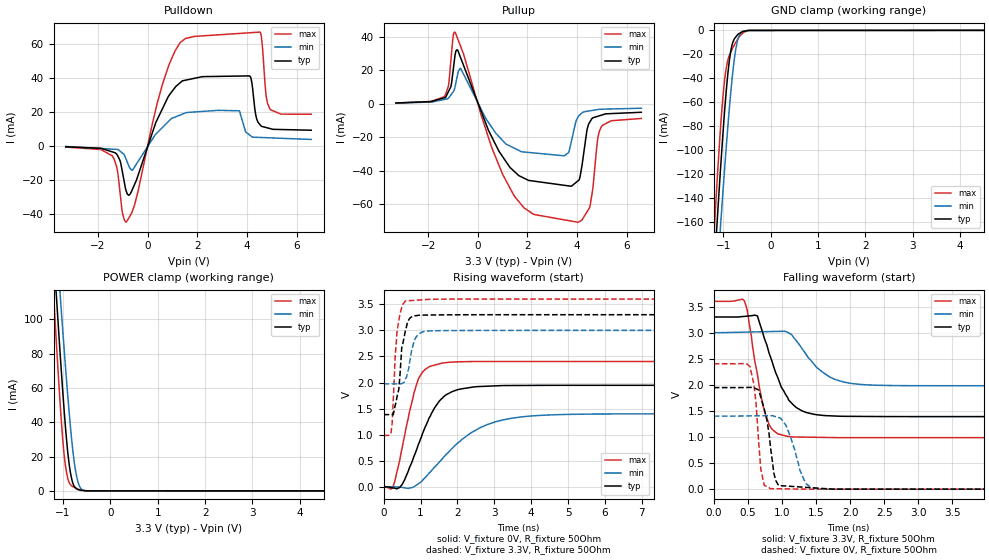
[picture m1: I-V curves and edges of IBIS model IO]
| Texas Instruments Incorporated
| 10-Channel Sequencer and System Health Monitor
| Marketing part#   Voltage Range   Package-type   #pins/pkg drawing
| UCD9090RGZR   3.0V - 3.6V   VQFN   48-pin  RGC
| UCD9090RGZT   3.0V - 3.6V   VQFN   48-pin  RGC
[IBIS ver]   4.0
[File name]   ucd9090.ibs
[File Rev]   1.0
[Date]   10/04/2016
[Source]   Simulations in SPECTRE
   Texas Instruments Incorporated.
   Analog-eLab, HPA
   12500 TI Blvd
   Dallas, TX -75243
   For Support e-mail: elab_ibis@list.ti.com
[Notes]   Revision History
   Rev 1.0: 10/04/2016
   - Initial version of the model
   - Model based on simulations from Spectre
   - Model not matched to measurements
   - Non-monotonic behavior is as per buffer simulations
   - Buffer [Model]s based on ucd9240.ibs Rev 1.1: 09/29/2010
[Disclaimer] This model is designed as an aid for customers of Texas Instruments.
 TI and its licensors and suppliers make no warranties, either expressed
 or implied, with respect to this  model, including the warranties of
 merchantability or fitness for a particular purpose.
 The model is provided solely on an "as is" basis. The entire risk as to
 its quality and performance is with the customer.
[Copyright] (C)Copyright 2016 Texas Instruments Incorporated.
   All rights reserved.
|   Component UCD9090RGZ
[Component]   UCD9090RGZ
[Manufacturer]  Texas Instruments Incorporated
[Package]   |48-pin VQFN package
|   typ   min   max
R_pkg   0.1229   0.0608   0.1600
L_pkg   1.8455n   1.2923n   2.3934n
C_pkg   0.1920p   0.1668p   0.2592p
[Pin] signal_name   model_name   R_pin   L_pin   C_pin
1   MON1   TERM   0.15085   2.25498n   0.20057p
2   MON2   TERM   0.13802   2.04542n   0.20645p
3   RESETN   TERM   0.12831   1.88923n   0.19375p
4   GPIO1   TERM   0.12256   1.79720n   0.17958p
5   GPIO2   TERM   0.13456   1.98873n   0.18502p
6   GPIO3   TERM   0.13010   1.91761n   0.19072p
7   GPIO4   TERM   0.12331   1.80911n   0.18509p
8   PMBUS_CLK   IO   0.12134   1.77773n   0.18285p
9   PMBUS_DATA   IO   0.12282   1.80149n   0.18453p
10   FPWM1_GPIO5  TERM   0.12680   1.86522n   0.18720p
11   FPWM2_GPIO6  TERM   0.13446   1.98842n   0.19728p
12   FPWM3_GPIO7  TERM   0.14463   2.15518n   0.18661p
13   FPWM4_GPIO8  TERM   0.14322   2.13188n   0.18595p
14   FPWM5_GPIO9  TERM   0.13149   1.93932n   0.19489p
15   FPWM6_GPIO10 TERM   0.12192   1.78462n   0.17983p
16   FPWM7_GPIO11 TERM   0.12141   1.77609n   0.17874p
17   FPWM8_GPIO12 TERM   0.11441   1.66343n   0.17498p
18   GPIO13   TERM   0.11107   1.60910n   0.16675p
19   PMBUS_ALERT  TERM   0.11356   1.64961n   0.17050p
20   PMBUS_CNTRL  TERM   0.11085   1.60523n   0.17438p
21   GPIO14   TERM   0.11338   1.64439n   0.17876p
22   PWM1_GP11   TERM   0.12108   1.76642n   0.18767p
23   PWM2_GP12   TERM   0.13231   1.94602n   0.20166p
24   GPIO15   TERM   0.14718   2.18768n   0.19313p
25   GPIO16   TERM   0.15035   2.23827n   0.19118p
26   GPIO17   GND   0.13904   2.05242n   0.20093p
27   TCK_GPIO18   TERM   0.13143   1.92932n   0.19435p
28   TDO_GPIO19   TERM   0.12400   1.80989n   0.18586p
29   TDI_GPIO20   TERM   0.12154   1.77043n   0.18272p
30   TMS_GPIO21   TERM   0.12231   1.78270n   0.18322p
31   TRSTN   TERM   0.12581   1.83871n   0.17867p
32   DVSS   GND   0.06081   1.33899n   0.22937p
33   V33D   POWER   0.06125   1.29229n   0.25072p
34   V33A   POWER   0.12567   1.83692n   0.19434p
35   BPCAP   TERM   0.06660   1.50738n   0.25918p
36   AVSS1   GND   0.14310   2.12168n   0.19030p
37   MON11   TERM   0.16000   2.39338n   0.20694p
38   MON3   TERM   0.14387   2.13082n   0.21646p
39   MON4   TERM   0.12997   1.90783n   0.19830p
40   MON5   TERM   0.11921   1.73650n   0.17853p
41   MON6   TERM   0.12377   1.80883n   0.17424p
42   MON7   TERM   0.12560   1.83791n   0.18459p
43   PMBUS_ADDR1  TERM   0.11624   1.68931n   0.18078p
44   PMBUS_ADDR0  TERM   0.11137   1.61293n   0.17532p
45   MON8   TERM   0.11165   1.61879n   0.17582p
46   MON9   TERM   0.11702   1.70582n   0.18487p
47   AVSS2   GND   0.06298   1.42062n   0.23983p
48   MON10   TERM   0.14809   2.20948n   0.19262p
[Model] TERM
Model_type Terminator
C_comp   0  0  0
| variable   typ   min   max
[Voltage Range]   3.30000V  3.00000V  3.60000V
[POWER Clamp Reference]  3.30000V  3.00000V  3.60000V
[GND Clamp Reference]   0.00000V  0.00000V  0.00000V
[Temperature Range]   27   110   -40
| Models and submodels in the file (2): TERM (Terminator), IO (I/O)
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|   IO 3.3V Model
[Model]   IO
Model_type   I/O
|Signals
Vinl =  0.65V
Vinh =  2.85V
Vmeas = 1.475V
Vref = 3.3V
|Rref = 50Ohm
| variable   typ   min   max
|C_comp Output Disabled   (NOM PVT)   (FAST PVT)   (SLOW PVT)
C_comp   1.475pF   1.443pF   1.508pF
|C_comp Output Low   (NOM PVT)   (SLOW PVT)   (FAST PVT)
|C_comp   2.352pF   2.12pF   2.485pF
|C_comp Output High   (NOM PVT)   (SLOW PVT)   (FAST PVT)
|C_comp   3.588pF   4.366pF   11.333pF
|Junction Temperature
[Temperature Range]   27.0   110.0   -40.0
[Voltage range]   3.3V   3.0V   3.6V
[pullup reference]   3.3V   3.0V   3.6V
[power clamp reference]   3.3V   3.0V   3.6V
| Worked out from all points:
|   slope of the pulldown table from 0 to 0.495 V, typ, clamps not added: 25.7 ohm
|   slope of the pullup table from 0 to 0.495 V, typ, clamps not added: 26.7 ohm
|   GND clamp passes 1 mA (typ) near -0.59 V on its own axis
|   POWER clamp passes 1 mA (typ) near -0.70 V on its own axis
|   falling waveform, V_fixture 3.3V, R_fixture 50Ohm: 20-80 % time 340ps typ, 421ps min, 207ps max; typ from 3.3 V to 1.39 V
|   rising waveform, V_fixture 0V, R_fixture 50Ohm: 20-80 % time 708ps typ, 1.32ns min, 449ps max; typ from 0 V to 1.95 V
|   rising waveform, V_fixture 3.3V, R_fixture 50Ohm: 20-80 % time 191ps typ, 179ps min, 136ps max; typ from 1.39 V to 3.3 V
|   falling waveform, V_fixture 0V, R_fixture 50Ohm: 20-80 % time 137ps typ, 200ps min, 87.7ps max; typ from 1.95 V to 0 V
[Pulldown]
|   Voltage   I(typ)   I(min)   I(max)
-3.3V     -501.7uA   -306.3uA   -648.9uA
-1.433V   -3.458mA   -1.887mA   -5.754mA
-867.3mV  -26.36mA   -7.887mA   -44.81mA
-598.8mV  -24.93mA   -13.94mA   -37.54mA
822.5mV   28.76mA    14.15mA    46.26mA
1.862V    39.67mA    19.93mA    64.32mA
3.681V    41.06mA    20.66mA    66.09mA
4.103V    41.15mA    6.486mA    66.49mA
4.526V    12.46mA    4.989mA    66.9mA
4.785V    10.76mA    4.84mA     28.27mA
4.923V    10.23mA    4.76mA     21.76mA
6.59V     9.23mA     3.797mA    18.61mA
[GND Clamp]
|   Voltage   I(typ)   I(min)   I(max)
-3.3V     -1.646A    -1.552A    -1.764A
-1.199V   -203.9mA   -245.2mA   -173.1mA
-1.164V   -181.5mA   -224.8mA   -148.7mA
-1.141V   -167.2mA   -211.4mA   -133.2mA
-1.119V   -153.7mA   -198.7mA   -119mA
-1.055V   -114.3mA   -162mA     -79.87mA
-952.2mV  -57.94mA   -105.5mA   -35.44mA
-847.3mV  -18.71mA   -54.52mA   -18.74mA
-733.4mV  -5.448mA   -15.18mA   -9.859mA
-669.8mV  -2.845mA   -4.95mA    -5.896mA
-590.3mV  -995.3uA   -1.043mA   -2.432mA
6.59V     0A         0A         0A
[Pullup]
|   Voltage   I(typ)   I(min)   I(max)
-3.3V     518.1uA    447.8uA    523.7uA
-1.363V   3.577mA    2.608mA    4.23mA
-1.19V    7.157mA    3.3mA      10.35mA
-932.3mV  27.47mA    9.295mA    42.97mA
-688.4mV  27.43mA    21.03mA    34.24mA
551.3mV   -19.46mA   -13.8mA    -25.62mA
1.43V     -39.88mA   -26.22mA   -54.12mA
3.485V    -48.74mA   -31.03mA   -69.42mA
4.008V    -46.42mA   -8.697mA   -70.8mA
4.508V    -11.06mA   -4.178mA   -62.05mA
4.98V     -6.738mA   -3.186mA   -13.6mA
6.59V     -5.03mA    -2.61mA    -8.729mA
[POWER Clamp]
|   Voltage   I(typ)   I(min)   I(max)
-3.3V     1.126A     1.059A     1.206A
-1.199V   139.3mA    169mA      114.3mA
-1.141V   114.2mA    146mA      86.88mA
-1.055V   77.88mA    112.5mA    48.83mA
-987.2mV  51.21mA    86.79mA    24.19mA
-947.1mV  36.9mA     72.18mA    14.51mA
-835.6mV  9.528mA    35.24mA    3.429mA
-759mV    2.557mA    16.12mA    2.066mA
-698.2mV  955.7uA    6.78mA     1.273mA
-621.5mV  370.3uA    1.374mA    619.3uA
-479.9mV  32.37uA    36uA       50.4uA
6.59V     0A         0A         0A
[Ramp]
R_load = 50
|   typ   min   max
dV/dt_r   1.16808/7.01565e-010  0.840176/1.30988e-009   1.44243/4.42526e-010
dV/dt_f   1.14541/3.06636e-010  0.610549/4.09332e-010   1.56775/2.07614e-010
[Falling Waveform]
V_fixture = 3.3V
V_fixture_min = 3V
V_fixture_max = 3.6V
R_fixture = 50Ohm
C_fixture = 0F
|   Time   V(typ)   V(min)   V(max)
0s        3.3V       3V         3.6V
450ps     3.312V     3.01V      3.608V
490ps     3.316V     3.011V     3.439V
640ps     3.321V     3.015V     2.204V
740ps     2.898V     3.018V     1.506V
850ps     2.466V     3.021V     1.156V
1.08ns    1.763V     3.008V     1.013V
1.61ns    1.412V     2.229V     991.8mV
2.22ns    1.394V     2.002V     987.3mV
14.98ns   1.391V     1.982V     987.1mV
[Rising Waveform]
V_fixture = 0V
V_fixture_min = 0V
V_fixture_max = 0V
R_fixture = 50Ohm
C_fixture = 0F
|   Time   V(typ)   V(min)   V(max)
|   0   1.02929e-009   2.40092e-009   7.786e-010
0s        443.4uV    408uV      455.8uV
270ps     -22.78mV   408uV      36.05mV
500ps     43.66mV    -10.02mV   738.4mV
700ps     368.1mV    -24.22mV   1.442V
940ps     810.1mV    58.93mV    2.065V
1.29ns    1.399V     306.5mV    2.317V
1.6ns     1.706V     544.1mV    2.375V
2.61ns    1.924V     1.131V     2.403V
3.93ns    1.944V     1.354V     2.404V
15ns      1.947V     1.4V       2.404V
[Rising Waveform]
V_fixture = 3.3V
V_fixture_min = 3V
V_fixture_max = 3.6V
R_fixture = 50Ohm
C_fixture = 0F
|   Time   V(typ)   V(min)   V(max)
0s        1.391V     1.982V     987.1mV
200ps     1.385V     1.974V     1.035V
230ps     1.385V     1.974V     1.214V
360ps     1.72V      1.974V     2.965V
410ps     1.867V     1.974V     3.18V
490ps     2.665V     1.981V     3.441V
590ps     2.997V     2.065V     3.564V
830ps     3.277V     2.807V     3.576V
1.17ns    3.293V     2.985V     3.592V
15ns      3.3V       3V         3.6V
[Falling Waveform]
|Gnd
V_fixture = 0V
V_fixture_min = 0V
V_fixture_max = 0V
R_fixture = 50Ohm
C_fixture = 0F
|   Time   V(typ)   V(min)   V(max)
0s        1.947V     1.4V       2.404V
530ps     1.95V      1.404V     2.35V
620ps     1.925V     1.406V     1.653V
690ps     1.759V     1.407V     382.1mV
830ps     822.2mV    1.409V     9.436mV
880ps     310.2mV    1.4V       8.565mV
950ps     70.21mV    1.374V     7.504mV
1.34ns    36.18mV    138mV      1mV
1.54ns    18.19mV    10.09mV    104.5uV
15ns      1.594nV    3.379nV    1.137nV
